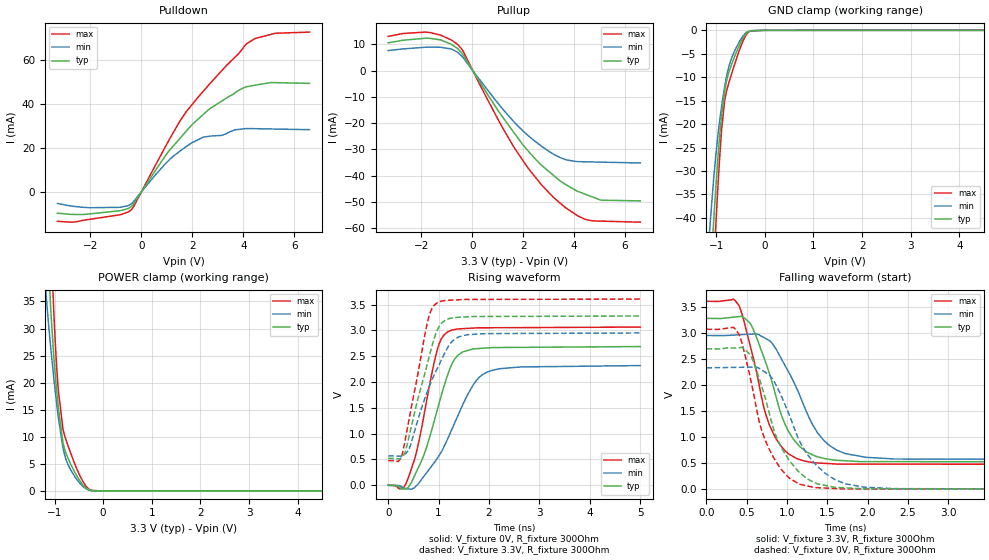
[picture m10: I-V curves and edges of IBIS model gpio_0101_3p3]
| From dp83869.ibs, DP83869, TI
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|   gpio_0101_3p3 Model
[Model]   gpio_0101_3p3
Model_type   I/O
Polarity   Non-Inverting
Enable   Active-Low
Vinl = 0.7
Vinh = 1.7
Vmeas = 1.65
Vref = 0
Cref = 2pF
Rref = 100000
|   typ   min   max
C_comp   1.10585pF   1.10585pF   1.45739pF
| Where Nom  PVT is Nominal Process, 3.3V,  27C
|   Fast PVT is Strong Process,  3.63V, -40C
|   Slow PVT is Weak Process,   2.97V, 125C
[Voltage Range]   3.3   2.97   3.63
|Junction Temperature
[Temperature Range]   27   125   -40
[Pullup Reference]   3.3   2.97   3.63
[Pulldown Reference]   0   -0   -0
[Power Clamp Reference]   3.3   2.97   3.63
[GND Clamp Reference]   0   0   0
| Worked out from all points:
|   slope of the pulldown table from 0 to 0.495 V, typ, clamps not added: 56.4 ohm
|   slope of the pullup table from 0 to 0.495 V, typ, clamps not added: 63.9 ohm
|   GND clamp passes 1 mA (typ) near -0.41 V on its own axis
|   POWER clamp passes 1 mA (typ) near -0.41 V on its own axis
|   falling waveform, V_fixture 3.3V, R_fixture 300Ohm: 20-80 % time 367ps typ, 457ps min, 314ps max; typ from 3.28 V to 0.523 V
|   rising waveform, V_fixture 0V, R_fixture 300Ohm: 20-80 % time 497ps typ, 701ps min, 377ps max; typ from 0 V to 2.69 V
|   rising waveform, V_fixture 3.3V, R_fixture 300Ohm: 20-80 % time 434ps typ, 555ps min, 360ps max; typ from 0.523 V to 3.28 V
|   falling waveform, V_fixture 0V, R_fixture 300Ohm: 20-80 % time 385ps typ, 453ps min, 334ps max; typ from 2.7 V to 0 V
[Pulldown]
|   Voltage   I(typ)   I(min)   I(max)
-3.3V     -9.718mA   -5.293mA   -13.4mA
-2.032V   -10.04mA   -7.226mA   -12.51mA
-824.7mV  -8.564mA   -7.032mA   -10.41mA
-414.8mV  -6.854mA   -5.596mA   -8.327mA
1.023V    17.77mA    13.76mA    22.28mA
1.489V    24.03mA    18.35mA    31.77mA
1.898V    29.46mA    21.7mA     38.43mA
2.69V     37.87mA    25.33mA    49.27mA
4.119V    47.85mA    28.83mA    67.33mA
4.469V    48.55mA    28.76mA    69.85mA
5.256V    49.72mA    28.6mA     72.19mA
6.6V      49.39mA    28.32mA    72.74mA
[GND Clamp]
|   Voltage   I(typ)   I(min)   I(max)
-3.3V     -489.2mA   -422.2mA   -556.8mA
-1.128V   -53.94mA   -41.75mA   -66.49mA
-1.053V   -40.94mA   -31.89mA   -50.85mA
-1.004V   -32.91mA   -26.23mA   -40.88mA
-914.8mV  -20.88mA   -18.15mA   -24.96mA
-886mV    -17.91mA   -16.01mA   -20.9mA
-824.7mV  -12.98mA   -11.96mA   -14.96mA
-737.5mV  -8.884mA   -7.637mA   -11.14mA
-632.6mV  -5.898mA   -4.664mA   -7.616mA
-450.4mV  -1.653mA   -1.242mA   -2.33mA
-360.4mV  -415.6uA   -340.7uA   -627.7uA
6.6V      0A         0A         0A
[Pullup]
|   Voltage   I(typ)   I(min)   I(max)
-3.3V     10.64mA    7.68mA     13.09mA
-1.746V   12.37mA    8.995mA    14.65mA
-1.228V   11.71mA    8.918mA    13.52mA
-600.9mV  8.648mA    7.203mA    10.24mA
-355.4mV  6.02mA     4.929mA    7.384mA
1.633V    -23.53mA   -19.45mA   -29.12mA
2.418V    -33.04mA   -26.57mA   -39.9mA
3.168V    -39.75mA   -31.69mA   -48.15mA
3.701V    -43.6mA    -34.05mA   -52.49mA
4.425V    -47.07mA   -34.75mA   -56.71mA
5.051V    -49.39mA   -34.88mA   -57.38mA
6.6V      -49.67mA   -35.2mA    -57.79mA
[POWER Clamp]
|   Voltage   I(typ)   I(min)   I(max)
-3.3V     592.7mA    473.7mA    711.1mA
-1.183V   53.33mA    37.6mA     74.54mA
-1.164V   49.45mA    35.35mA    69.48mA
-1.121V   40.99mA    30.62mA    58.01mA
-1.071V   32.56mA    25.84mA    45.66mA
-1.013V   24.62mA    20.7mA     32.69mA
-952.4mV  18.17mA    15.83mA    22.43mA
-922.7mV  15.44mA    13.63mA    18.69mA
-824.7mV  8.834mA    7.855mA    11.3mA
-669.2mV  4.995mA    3.928mA    7.01mA
-332.6mV  387.6uA    312.9uA    668.4uA
6.6V      0A         0A         0A
[Ramp]
R_load = 300
|   typ   min   max
dV/dt_r   1.61298/4.94909e-10   1.39173/6.98918e-10   1.83963/3.75895e-10
dV/dt_f   1.65485/3.63801e-10   1.42877/4.54482e-10   1.87931/3.11031e-10
[Falling Waveform]
V_fixture = 3.3V
V_fixture_min = 2.97V
V_fixture_max = 3.63V
R_fixture = 300Ohm
C_fixture = 0F
|   Time   V(typ)   V(min)   V(max)
0s        3.281V     2.952V     3.609V
357ps     3.307V     2.962V     3.622V
430.1ps   3.318V     2.968V     3.419V
542.2ps   3.188V     2.978V     2.759V
787.5ps   2.189V     2.848V     1.209V
951.8ps   1.333V     2.442V     780.5mV
1.121ns   882.9mV    1.932V     587.4mV
1.391ns   618.4mV    1.058V     502.3mV
1.731ns   545.1mV    681.4mV    482.1mV
5ns       522.7mV    570.8mV    476.8mV
[Rising Waveform]
V_fixture = 0V
V_fixture_min = 0V
V_fixture_max = 0V
R_fixture = 300Ohm
C_fixture = 0F
|   Time   V(typ)   V(min)   V(max)
0s        273.9uV    407.9uV    284uV
235.9ps   -46.35mV   -10.78mV   -69.15mV
387.5ps   -48.6mV    -69.57mV   117.7mV
605.2ps   356.9mV    40.88mV    835.2mV
967.6ps   1.441V     515.4mV    2.609V
1.171ns   2.116V     884.2mV    2.968V
1.466ns   2.578V     1.534V     3.034V
1.738ns   2.647V     2.019V     3.05V
1.974ns   2.663V     2.198V     3.052V
5ns       2.689V     2.32V      3.066V
[Rising Waveform]
V_fixture = 3.3V
V_fixture_min = 2.97V
V_fixture_max = 3.63V
R_fixture = 300Ohm
C_fixture = 0F
|   Time   V(typ)   V(min)   V(max)
0s        522.7mV    570.9mV    476.8mV
195.6ps   514.6mV    566.3mV    460.8mV
277.5ps   551.2mV    570.1mV    597.5mV
409.5ps   929.6mV    688.6mV    1.259V
780.7ps   2.372V     1.829V     3.17V
856.6ps   2.655V     2.014V     3.405V
963.3ps   2.987V     2.244V     3.532V
1.23ns    3.236V     2.747V     3.587V
1.582ns   3.266V     2.919V     3.601V
5ns       3.281V     2.952V     3.609V
[Falling Waveform]
|Gnd
V_fixture = 0V
V_fixture_min = 0V
V_fixture_max = 0V
R_fixture = 300Ohm
C_fixture = 0F
|   Time   V(typ)   V(min)   V(max)
0s        2.696V     2.331V     3.072V
353.9ps   2.713V     2.339V     3.082V
537.4ps   2.591V     2.344V     2.182V
657.6ps   2.117V     2.317V     1.282V
780.7ps   1.453V     2.194V     763.3mV
923.5ps   814.3mV    1.809V     392.5mV
1.153ns   324.6mV    932.2mV    96.96mV
1.474ns   71.88mV    304.2mV    21.8mV
1.956ns   8.347mV    39.43mV    5.744mV
5ns       266.6uV    387.7uV    280.2uV
